ORGANIZATION_BLOCK OB 1
BEGIN

	// Check instance-DB length
	AUF		DB 1
	L		DBLG
	__ASSERT==	__ACCU 1,	10
	AUF		DB 0


	// Check Preset
	CALL	SFB 1, DB 1 (
		CD	:= TRUE,
		LOAD	:= TRUE,
		PV	:= 2,
		Q	:= M 0.0,
		CV	:= MW 2,
	)
	L		MW 2
	__ASSERT==	__ACCU 1,	2
	U		M 0.0
	__ASSERT==	__STW VKE,	0
	U		DB1.DBX 8.0	// CDO
	__ASSERT==	__STW VKE,	1

	CALL	SFB 1, DB 1 (
		CD	:= FALSE,
		LOAD	:= TRUE,
		PV	:= -2,
		Q	:= M 0.0,
		CV	:= MW 2,
	)
	L		MW 2
	__ASSERT==	__ACCU 1,	-2
	U		M 0.0
	__ASSERT==	__STW VKE,	1
	U		DB1.DBX 8.0	// CDO
	__ASSERT==	__STW VKE,	0

	CALL	SFB 1, DB 1 (
		CD	:= TRUE,
		LOAD	:= TRUE,
		PV	:= 2,
		Q	:= M 0.0,
		CV	:= MW 2,
	)
	L		MW 2
	__ASSERT==	__ACCU 1,	2
	U		M 0.0
	__ASSERT==	__STW VKE,	0
	U		DB1.DBX 8.0	// CDO
	__ASSERT==	__STW VKE,	1

	CALL	SFB 1, DB 1 (
		CD	:= FALSE,
		LOAD	:= FALSE,
		PV	:= 0,
		Q	:= M 0.0,
		CV	:= MW 2,
	)
	L		MW 2
	__ASSERT==	__ACCU 1,	2
	U		M 0.0
	__ASSERT==	__STW VKE,	0
	U		DB1.DBX 8.0	// CDO
	__ASSERT==	__STW VKE,	0


	// Test CTD counter
	CALL	SFB 1, DB 1 (
		CD	:= FALSE,
		LOAD	:= FALSE,
		PV	:= 10,
		Q	:= M 0.0,
		CV	:= MW 2,
	)
	L		MW 2
	__ASSERT==	__ACCU 1,	2
	U		M 0.0
	__ASSERT==	__STW VKE,	0
	U		DB1.DBX 8.0	// CDO
	__ASSERT==	__STW VKE,	0

	CALL	SFB 1, DB 1 (
		CD	:= FALSE,
		LOAD	:= FALSE,
		PV	:= 10,
		Q	:= M 0.0,
		CV	:= MW 2,
	)
	L		MW 2
	__ASSERT==	__ACCU 1,	2
	U		M 0.0
	__ASSERT==	__STW VKE,	0
	U		DB1.DBX 8.0	// CDO
	__ASSERT==	__STW VKE,	0

	CALL	SFB 1, DB 1 (
		CD	:= TRUE,
		LOAD	:= FALSE,
		PV	:= 10,
		Q	:= M 0.0,
		CV	:= MW 2,
	)
	L		MW 2
	__ASSERT==	__ACCU 1,	1
	U		M 0.0
	__ASSERT==	__STW VKE,	0
	U		DB1.DBX 8.0	// CDO
	__ASSERT==	__STW VKE,	1

	CALL	SFB 1, DB 1 (
		CD	:= FALSE,
		LOAD	:= FALSE,
		PV	:= 10,
		Q	:= M 0.0,
		CV	:= MW 2,
	)
	L		MW 2
	__ASSERT==	__ACCU 1,	1
	U		M 0.0
	__ASSERT==	__STW VKE,	0
	U		DB1.DBX 8.0	// CDO
	__ASSERT==	__STW VKE,	0

	CALL	SFB 1, DB 1 (
		CD	:= TRUE,
		LOAD	:= FALSE,
		PV	:= 10,
		Q	:= M 0.0,
		CV	:= MW 2,
	)
	L		MW 2
	__ASSERT==	__ACCU 1,	0
	U		M 0.0
	__ASSERT==	__STW VKE,	1
	U		DB1.DBX 8.0	// CDO
	__ASSERT==	__STW VKE,	1

	CALL	SFB 1, DB 1 (
		CD	:= FALSE,
		LOAD	:= FALSE,
		PV	:= 10,
		Q	:= M 0.0,
		CV	:= MW 2,
	)
	L		MW 2
	__ASSERT==	__ACCU 1,	0
	U		M 0.0
	__ASSERT==	__STW VKE,	1
	U		DB1.DBX 8.0	// CDO
	__ASSERT==	__STW VKE,	0

	CALL	SFB 1, DB 1 (
		CD	:= TRUE,
		LOAD	:= FALSE,
		PV	:= 10,
		Q	:= M 0.0,
		CV	:= MW 2,
	)
	L		MW 2
	__ASSERT==	__ACCU 1,	-1
	U		M 0.0
	__ASSERT==	__STW VKE,	1
	U		DB1.DBX 8.0	// CDO
	__ASSERT==	__STW VKE,	1

	CALL	SFB 1, DB 1 (
		CD	:= FALSE,
		LOAD	:= FALSE,
		PV	:= 10,
		Q	:= M 0.0,
		CV	:= MW 2,
	)
	L		MW 2
	__ASSERT==	__ACCU 1,	-1
	U		M 0.0
	__ASSERT==	__STW VKE,	1
	U		DB1.DBX 8.0	// CDO
	__ASSERT==	__STW VKE,	0

	CALL	SFB 1, DB 1 (
		CD	:= TRUE,
		LOAD	:= FALSE,
		PV	:= 10,
		Q	:= M 0.0,
		CV	:= MW 2,
	)
	L		MW 2
	__ASSERT==	__ACCU 1,	-2
	U		M 0.0
	__ASSERT==	__STW VKE,	1
	U		DB1.DBX 8.0	// CDO
	__ASSERT==	__STW VKE,	1

	CALL	SFB 1, DB 1 (
		CD	:= FALSE,
		LOAD	:= FALSE,
		PV	:= 10,
		Q	:= M 0.0,
		CV	:= MW 2,
	)
	L		MW 2
	__ASSERT==	__ACCU 1,	-2
	U		M 0.0
	__ASSERT==	__STW VKE,	1
	U		DB1.DBX 8.0	// CDO
	__ASSERT==	__STW VKE,	0


	// Test limit
	L		-32767
	T		DB1.DBW 6	// CV

	CALL	SFB 1, DB 1 (
		CD	:= FALSE,
		LOAD	:= FALSE,
		PV	:= 0,
		Q	:= M 0.0,
		CV	:= MW 2,
	)
	L		MW 2
	__ASSERT==	__ACCU 1,	-32767
	U		M 0.0
	__ASSERT==	__STW VKE,	1
	U		DB1.DBX 8.0	// CDO
	__ASSERT==	__STW VKE,	0

	CALL	SFB 1, DB 1 (
		CD	:= TRUE,
		LOAD	:= FALSE,
		PV	:= 0,
		Q	:= M 0.0,
		CV	:= MW 2,
	)
	L		MW 2
	__ASSERT==	__ACCU 1,	-32768
	U		M 0.0
	__ASSERT==	__STW VKE,	1
	U		DB1.DBX 8.0	// CDO
	__ASSERT==	__STW VKE,	1

	CALL	SFB 1, DB 1 (
		CD	:= FALSE,
		LOAD	:= FALSE,
		PV	:= 0,
		Q	:= M 0.0,
		CV	:= MW 2,
	)
	L		MW 2
	__ASSERT==	__ACCU 1,	-32768
	U		M 0.0
	__ASSERT==	__STW VKE,	1
	U		DB1.DBX 8.0	// CDO
	__ASSERT==	__STW VKE,	0

	CALL	SFB 1, DB 1 (
		CD	:= TRUE,
		LOAD	:= FALSE,
		PV	:= 0,
		Q	:= M 0.0,
		CV	:= MW 2,
	)
	L		MW 2
	__ASSERT==	__ACCU 1,	-32768
	U		M 0.0
	__ASSERT==	__STW VKE,	1
	U		DB1.DBX 8.0	// CDO
	__ASSERT==	__STW VKE,	1

	CALL	SFB 1, DB 1 (
		CD	:= FALSE,
		LOAD	:= FALSE,
		PV	:= 0,
		Q	:= M 0.0,
		CV	:= MW 2,
	)
	L		MW 2
	__ASSERT==	__ACCU 1,	-32768
	U		M 0.0
	__ASSERT==	__STW VKE,	1
	U		DB1.DBX 8.0	// CDO
	__ASSERT==	__STW VKE,	0

	CALL	SFB 1, DB 1 (
		CD	:= TRUE,
		LOAD	:= FALSE,
		PV	:= 0,
		Q	:= M 0.0,
		CV	:= MW 2,
	)
	L		MW 2
	__ASSERT==	__ACCU 1,	-32768
	U		M 0.0
	__ASSERT==	__STW VKE,	1
	U		DB1.DBX 8.0	// CDO
	__ASSERT==	__STW VKE,	1

	CALL	SFB 1, DB 1 (
		CD	:= FALSE,
		LOAD	:= TRUE,
		PV	:= 10,
		Q	:= M 0.0,
		CV	:= MW 2,
	)
	L		MW 2
	__ASSERT==	__ACCU 1,	10
	U		M 0.0
	__ASSERT==	__STW VKE,	0
	U		DB1.DBX 8.0	// CDO
	__ASSERT==	__STW VKE,	0


END_ORGANIZATION_BLOCK


DATA_BLOCK DB 1
	SFB 1
BEGIN
END_DATA_BLOCK
